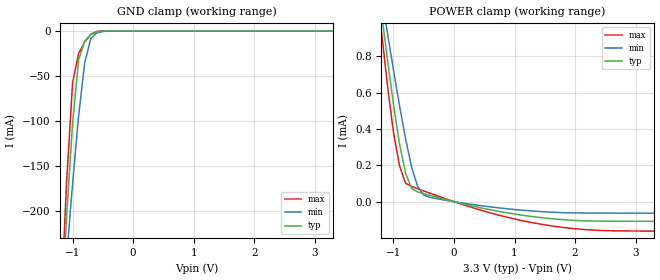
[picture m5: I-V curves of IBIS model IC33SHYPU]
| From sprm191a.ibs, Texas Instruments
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[Model]   IC33SHYPU
Model_type   Input
Polarity   Non-Inverting
| signals   A, Y
Vinl = 0.8V
Vinh = 2.0V
|   typ   min   max
C_comp   1.4592p   1.4336p   1.5063p
|   typ   min   max
[Temperature Range]   25   -40   125
|   typ   min   max
[Voltage Range]   3.30V   3.00V   3.60V
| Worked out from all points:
|   GND clamp passes 1 mA (typ) near -0.61 V on its own axis
|   POWER clamp passes 1 mA (typ) near -1.18 V on its own axis
[GND_clamp]
|   Voltage   I(typ)   I(min)   I(max)
-3.3V     -3.046A    -2.3A      -3.955A
-1.2V     -324.1mA   -338.8mA   -319.7mA
-1.1V     -207.5mA   -252.5mA   -169.7mA
-1V       -102.7mA   -169.8mA   -57.61mA
-900mV    -31.8mA    -94.42mA   -24.95mA
-800mV    -11.42mA   -35.62mA   -12.07mA
-700mV    -4.192mA   -8.508mA   -3.56mA
-600mV    -819.1uA   -2.049mA   -409.8uA
-500mV    -75.22uA   -368.2uA   -19.35uA
-400mV    -4.217uA   -45.05uA   -434.7nA
3.3V      222pA      35.04nA    133.2pA
[POWER_clamp]
|   Voltage   I(typ)   I(min)   I(max)
-3.3V     6.905mA    5.744mA    7.841mA
-1.2V     1.047mA    1.139mA    943.6uA
-1.1V     786.2uA    930.8uA    644.3uA
-1V       537.8uA    726.9uA    382uA
-900mV    318.6uA    530.3uA    198.8uA
-800mV    158.1uA    346.8uA    101.7uA
-700mV    72.97uA    190.9uA    83uA
-600mV    53.62uA    83.38uA    70.93uA
-500mV    44.09uA    36.26uA    58.94uA
500mV     -38.02uA   -24.54uA   -52.48uA
1.4V      -86.44uA   -53.97uA   -122uA
3.3V      -108.3uA   -63.63uA   -162uA
